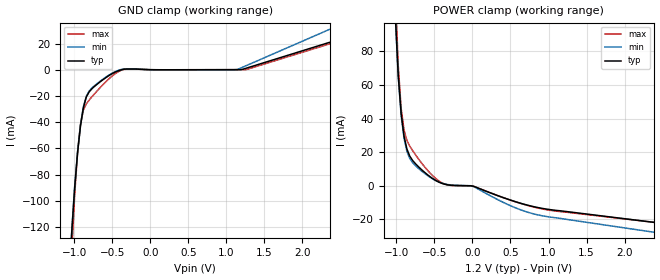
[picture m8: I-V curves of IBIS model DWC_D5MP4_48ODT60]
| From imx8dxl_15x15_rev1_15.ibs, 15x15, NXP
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[Model] DWC_D5MP4_48ODT60
Model_type   Input
Polarity   Non-Inverting
Enable   Active-High
C_comp   1.348pF   1.271pF   1.374pF
C_comp_power_clamp   335.985fF   329.909fF   346.315fF
C_comp_gnd_clamp 1.002pF   926.265fF   1.019pF
Vinh = 960.000mV
Vinl = 774.000mV
[Model Spec]
D_overshoot_ampl_h 0.4 NA   NA
D_overshoot_ampl_l 0.4 NA   NA
D_overshoot_area_l 60.000p NA   NA
D_overshoot_area_h 60.000p NA   NA
[Receiver Thresholds]
Vth = 867.000mV
Vth_min = 855.000mV
Vth_max = 879.000mV
Vinh_ac = 68.000mV
Vinh_dc = 68.000mV
Vinl_ac = -68.000mV
Vinl_dc = -68.000mV
Tslew_ac = 5.000ns
Reference_supply Power_clamp_ref
[Temperature Range]   25.000   125.000   -40.000
[Voltage Range]   1.200V   1.140V   1.260V
[GND Clamp Reference]   0.00V   0.00V   0.00V
[C Comp Corner]
| variable   typ   min   max
C_comp 1.348pF   1.374pF   1.271pF
C_comp_pullup 335.985fF   346.315fF   329.909fF
C_comp_pulldown 1.002pF   1.019pF   926.265fF
[POWER Clamp Reference]   1.200V   1.140V   1.260V
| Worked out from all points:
|   GND clamp passes 1 mA (typ) near -0.43 V on its own axis
|   POWER clamp passes 1 mA (typ) near -0.37 V on its own axis
[GND Clamp]
-1.184V   -337.6mA   -336.6mA   -426mA
-1.031V   -123.5mA   -122.6mA   -138.8mA
-992.7mV  -89.64mA   -88.76mA   -95.17mA
-954.5mV  -62.99mA   -62.21mA   -62.91mA
-916.4mV  -42.74mA   -42.01mA   -41.49mA
-878.2mV  -28.78mA   -28.09mA   -30.64mA
-840mV    -20.8mA    -20.16mA   -25.99mA
-763.6mV  -14.32mA   -13.75mA   -20.45mA
-610.9mV  -7.16mA    -6.714mA   -10.77mA
-343.6mV  433.7uA    670.6uA    344.7uA
1.145V    65.57uA    178.2uA    78.74uA
2.367V    21.07mA    31.04mA    19.89mA
[Power Clamp]
-1.167V   361.5mA    358.4mA    466.1mA
-1.015V   102.2mA    101.3mA    116.4mA
-976.4mV  66.14mA    65.36mA    71.85mA
-938.2mV  43.23mA    42.17mA    46.26mA
-900mV    29.57mA    28.32mA    33.24mA
-861.8mV  21.84mA    20.48mA    27.01mA
-785.5mV  15mA       13.7mA     20.84mA
-556.4mV  5.379mA    5.034mA    7.521mA
-365.5mV  940uA      1.097mA    1.059mA
16.4mV    -300.7uA   -473.9uA   -294.9uA
856.4mV   -12.91mA   -17.27mA   -13.18mA
2.384V    -21.73mA   -27.61mA   -21.72mA
